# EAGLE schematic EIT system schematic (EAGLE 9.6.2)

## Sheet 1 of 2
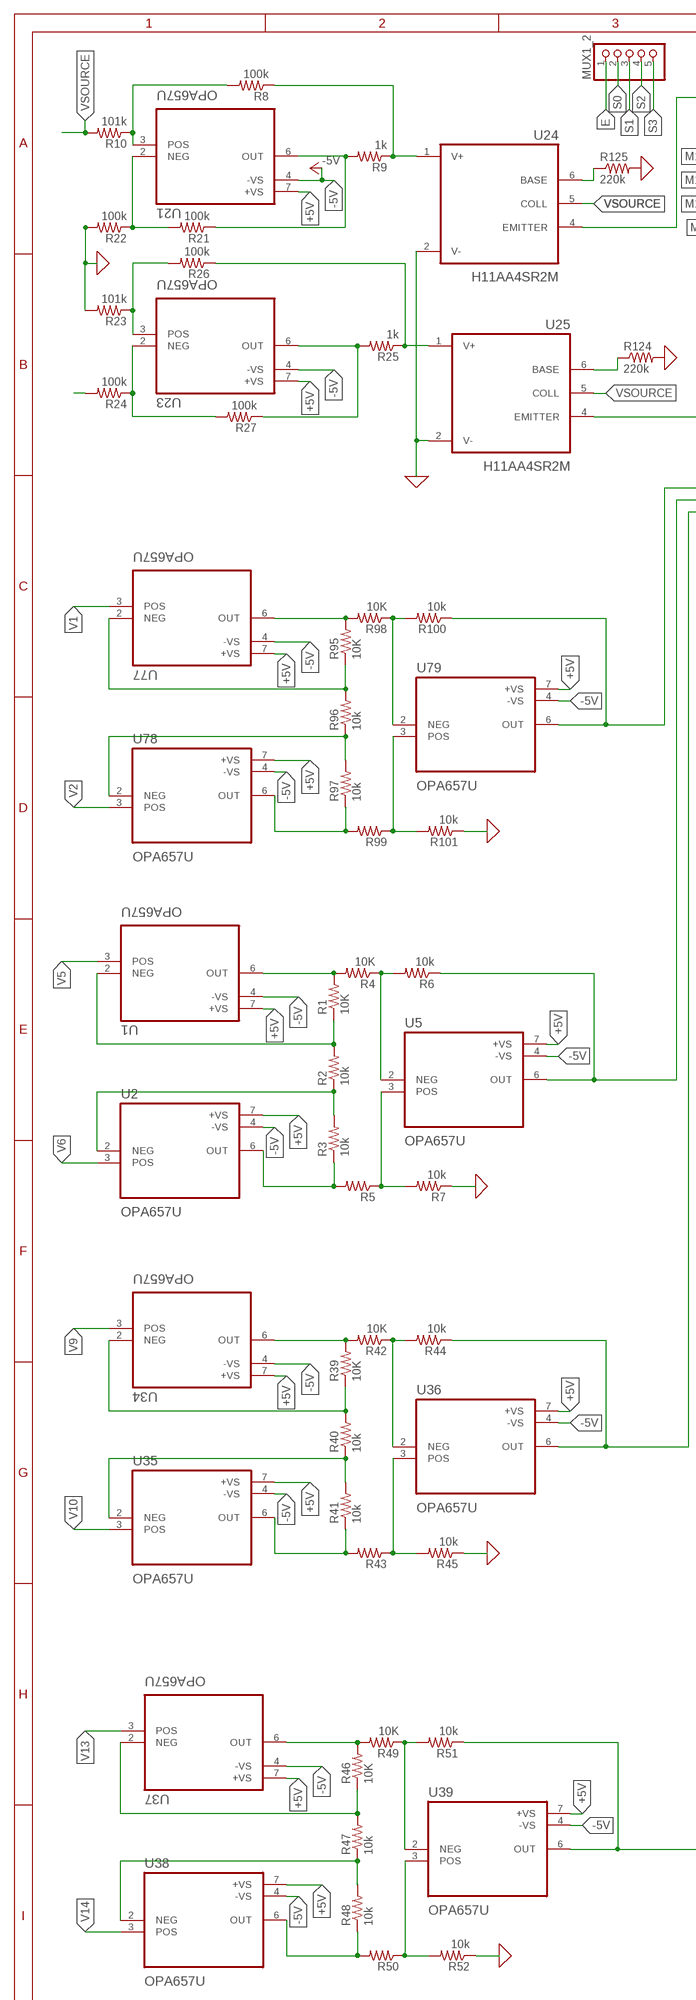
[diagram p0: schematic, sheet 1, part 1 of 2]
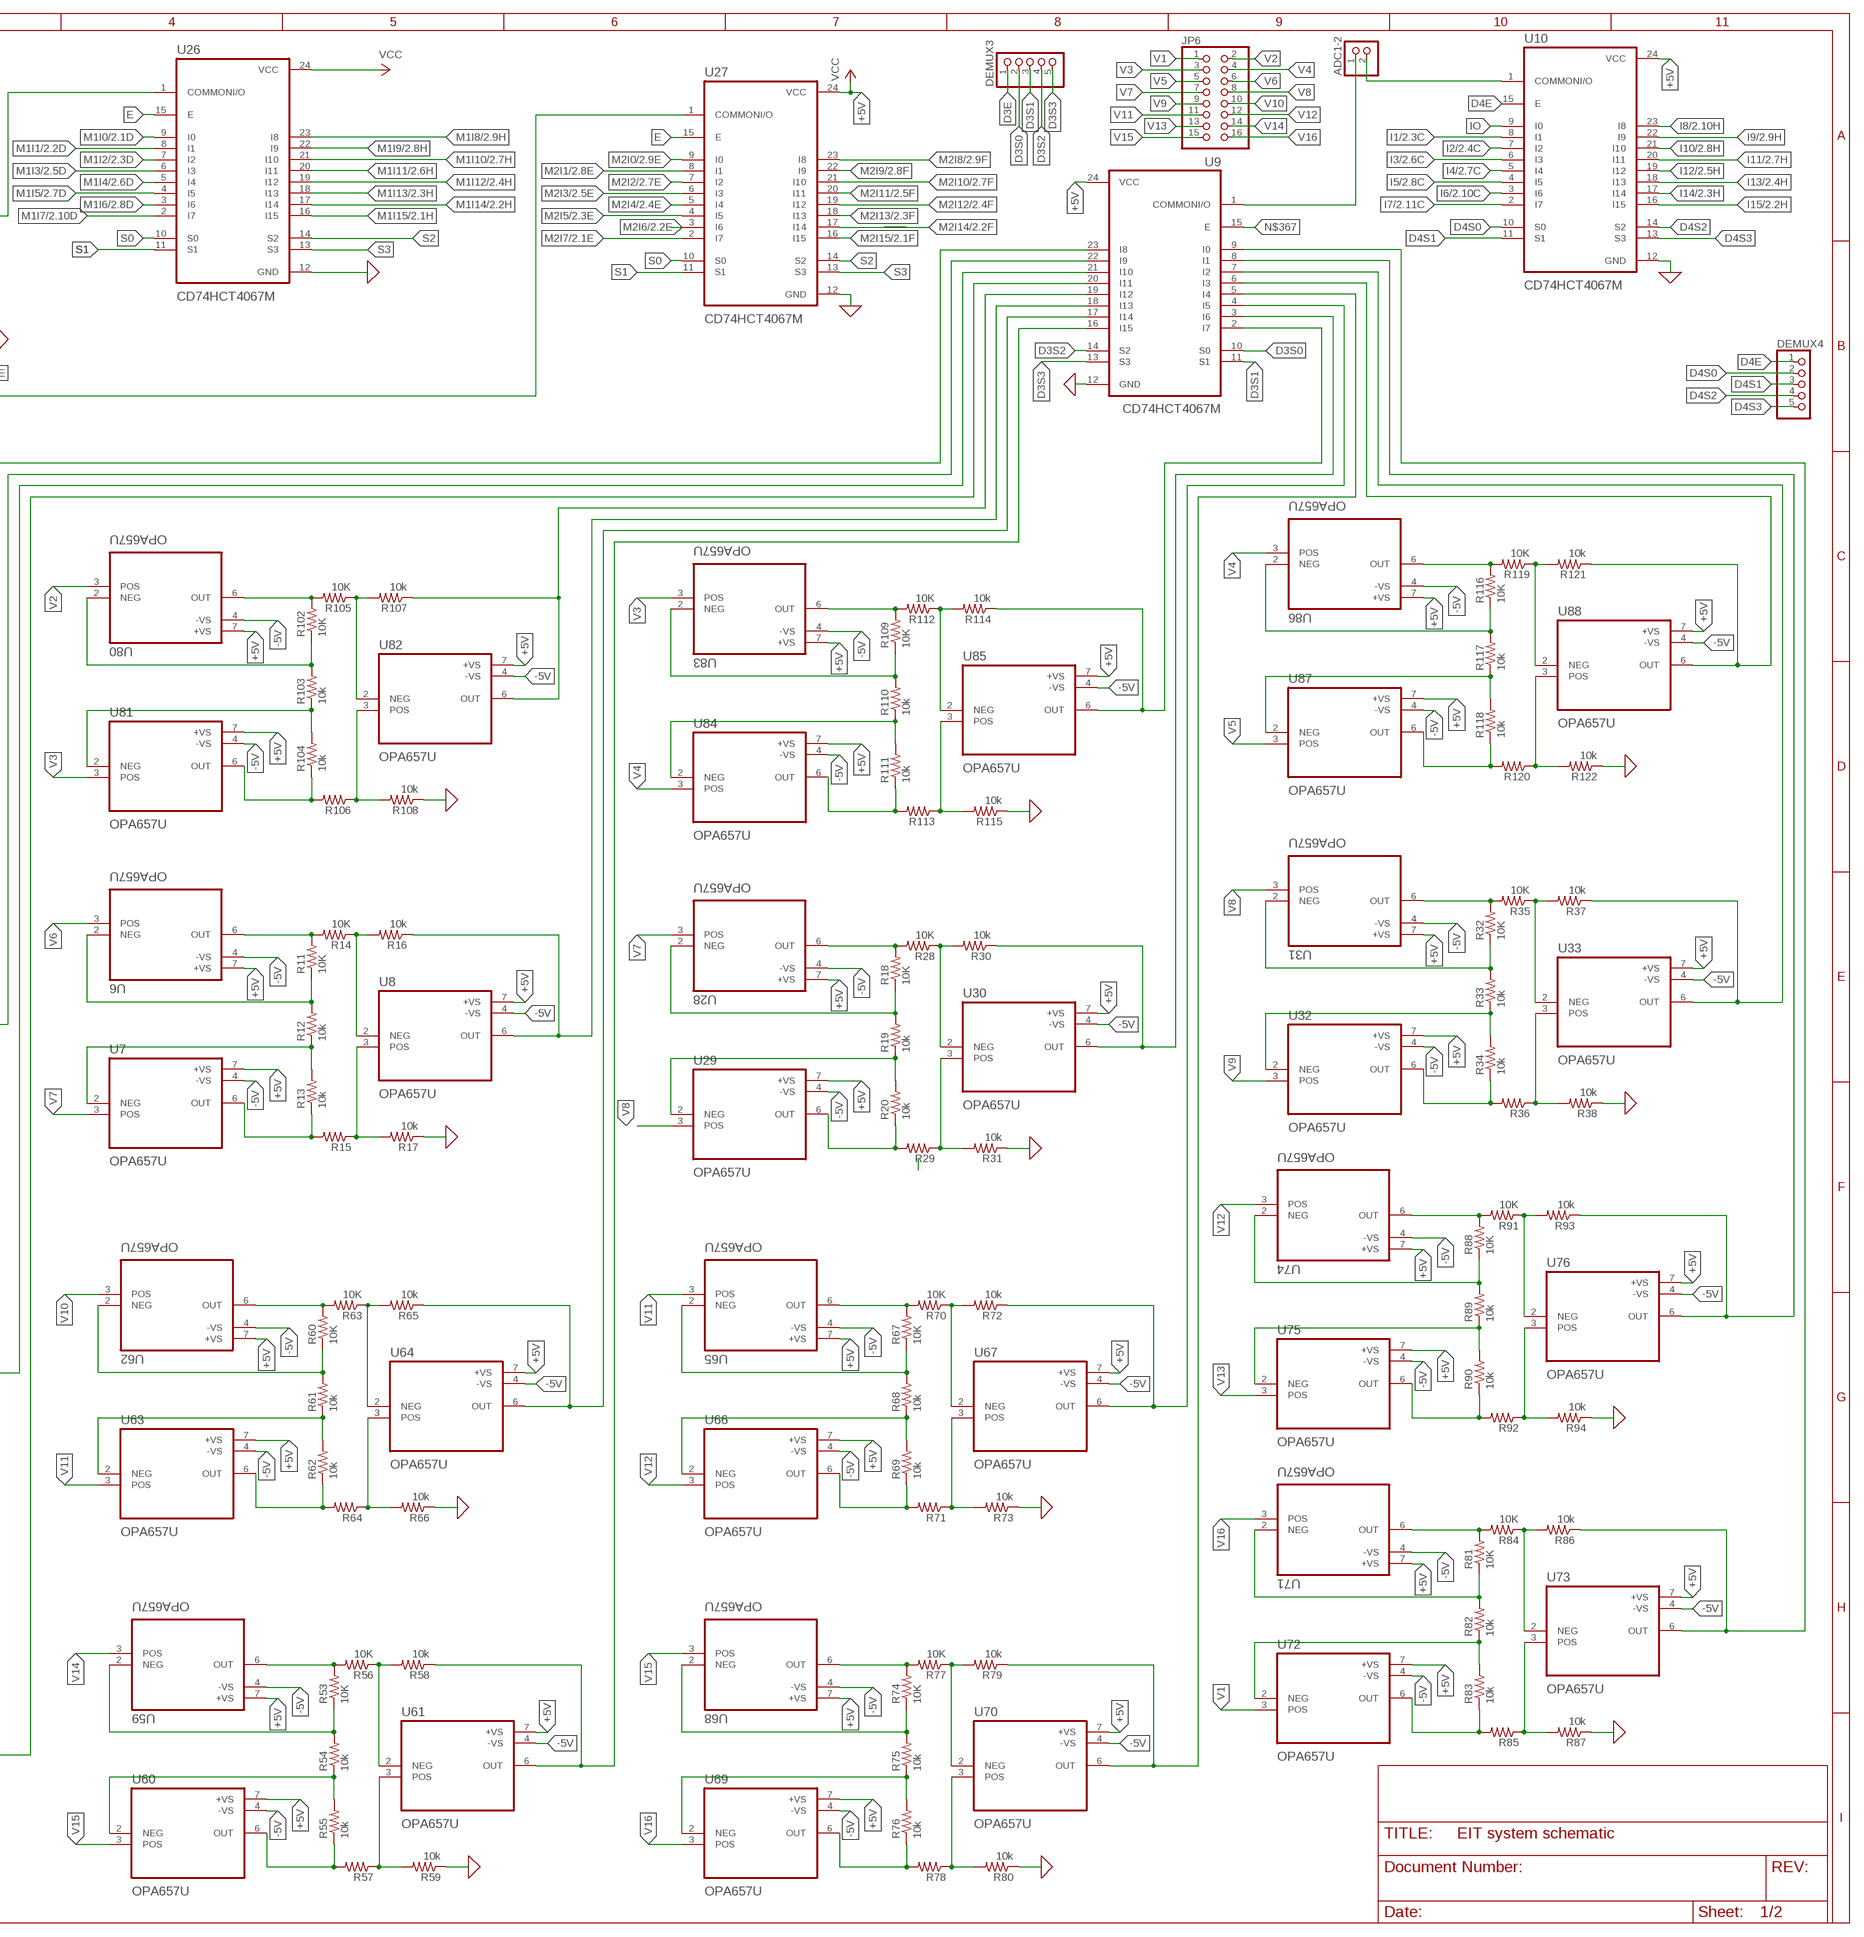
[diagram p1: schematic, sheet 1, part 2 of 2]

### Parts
ADC1-2  PINHD-1X2  [1X02]
DEMUX3  PINHD-1X5  [1X05]
DEMUX4  PINHD-1X5  [1X05]
JP6  PINHD-2X8  [2X08]
MUX1_2  PINHD-1X55X2MM  [1_05X2MM]
R1  10K  R-US_M0805  [M0805]
R2  10k  R-US_M0805  [M0805]
R3  10k  R-US_M0805  [M0805]
R4  10K  R-US_M0805  [M0805]
R5  R-US_M0805  [M0805]
R6  10k  R-US_M0805  [M0805]
R7  10k  R-US_M0805  [M0805]
R8  100k  R-US_M0805  [M0805]
R9  1k  R-US_M0805  [M0805]
R10  101k  R-US_M0805  [M0805]
R11  10K  R-US_M0805  [M0805]
R12  10k  R-US_M0805  [M0805]
R13  10k  R-US_M0805  [M0805]
R14  10K  R-US_M0805  [M0805]
R15  R-US_M0805  [M0805]
R16  10k  R-US_M0805  [M0805]
R17  10k  R-US_M0805  [M0805]
R18  10K  R-US_M0805  [M0805]
R19  10k  R-US_M0805  [M0805]
R20  10k  R-US_M0805  [M0805]
R21  100k  R-US_M0805  [M0805]
R22  100k  R-US_M0805  [M0805]
R23  101k  R-US_M0805  [M0805]
R24  100k  R-US_M0805  [M0805]
R25  1k  R-US_M0805  [M0805]
R26  100k  R-US_M0805  [M0805]
R27  100k  R-US_M0805  [M0805]
R28  10K  R-US_M0805  [M0805]
R29  R-US_M0805  [M0805]
R30  10k  R-US_M0805  [M0805]
R31  10k  R-US_M0805  [M0805]
R32  10K  R-US_M0805  [M0805]
R33  10k  R-US_M0805  [M0805]
R34  10k  R-US_M0805  [M0805]
R35  10K  R-US_M0805  [M0805]
R36  R-US_M0805  [M0805]
R37  10k  R-US_M0805  [M0805]
R38  10k  R-US_M0805  [M0805]
R39  10K  R-US_M0805  [M0805]
R40  10k  R-US_M0805  [M0805]
R41  10k  R-US_M0805  [M0805]
R42  10K  R-US_M0805  [M0805]
R43  R-US_M0805  [M0805]
R44  10k  R-US_M0805  [M0805]
R45  10k  R-US_M0805  [M0805]
R46  10K  R-US_M0805  [M0805]
R47  10k  R-US_M0805  [M0805]
R48  10k  R-US_M0805  [M0805]
R49  10K  R-US_M0805  [M0805]
R50  R-US_M0805  [M0805]
R51  10k  R-US_M0805  [M0805]
R52  10k  R-US_M0805  [M0805]
R53  10K  R-US_M0805  [M0805]
R54  10k  R-US_M0805  [M0805]
R55  10k  R-US_M0805  [M0805]
R56  10K  R-US_M0805  [M0805]
R57  R-US_M0805  [M0805]
R58  10k  R-US_M0805  [M0805]
R59  10k  R-US_M0805  [M0805]
R60  10K  R-US_M0805  [M0805]
R61  10k  R-US_M0805  [M0805]
R62  10k  R-US_M0805  [M0805]
R63  10K  R-US_M0805  [M0805]
R64  R-US_M0805  [M0805]
R65  10k  R-US_M0805  [M0805]
R66  10k  R-US_M0805  [M0805]
R67  10K  R-US_M0805  [M0805]
R68  10k  R-US_M0805  [M0805]
R69  10k  R-US_M0805  [M0805]
R70  10K  R-US_M0805  [M0805]
R71  R-US_M0805  [M0805]
R72  10k  R-US_M0805  [M0805]
R73  10k  R-US_M0805  [M0805]
R74  10K  R-US_M0805  [M0805]
R75  10k  R-US_M0805  [M0805]
R76  10k  R-US_M0805  [M0805]
R77  10K  R-US_M0805  [M0805]
R78  R-US_M0805  [M0805]
R79  10k  R-US_M0805  [M0805]
R80  10k  R-US_M0805  [M0805]
R81  10K  R-US_M0805  [M0805]
R82  10k  R-US_M0805  [M0805]
R83  10k  R-US_M0805  [M0805]
R84  10K  R-US_M0805  [M0805]
R85  R-US_M0805  [M0805]
R86  10k  R-US_M0805  [M0805]
R87  10k  R-US_M0805  [M0805]
R88  10K  R-US_M0805  [M0805]
R89  10k  R-US_M0805  [M0805]
R90  10k  R-US_M0805  [M0805]
R91  10K  R-US_M0805  [M0805]
R92  R-US_M0805  [M0805]
R93  10k  R-US_M0805  [M0805]
R94  10k  R-US_M0805  [M0805]
R95  10K  R-US_M0805  [M0805]
R96  10k  R-US_M0805  [M0805]
R97  10k  R-US_M0805  [M0805]
R98  10K  R-US_M0805  [M0805]
R99  R-US_M0805  [M0805]
R100  10k  R-US_M0805  [M0805]
R101  10k  R-US_M0805  [M0805]
R102  10K  R-US_M0805  [M0805]
R103  10k  R-US_M0805  [M0805]
R104  10k  R-US_M0805  [M0805]
R105  10K  R-US_M0805  [M0805]
R106  R-US_M0805  [M0805]
R107  10k  R-US_M0805  [M0805]
R108  10k  R-US_M0805  [M0805]
R109  10K  R-US_M0805  [M0805]
R110  10k  R-US_M0805  [M0805]
R111  10k  R-US_M0805  [M0805]
R112  10K  R-US_M0805  [M0805]
R113  R-US_M0805  [M0805]
R114  10k  R-US_M0805  [M0805]
R115  10k  R-US_M0805  [M0805]
R116  10K  R-US_M0805  [M0805]
R117  10k  R-US_M0805  [M0805]
R118  10k  R-US_M0805  [M0805]
R119  10K  R-US_M0805  [M0805]
R120  R-US_M0805  [M0805]
R121  10k  R-US_M0805  [M0805]
R122  10k  R-US_M0805  [M0805]
R124  220k  R-US_M0805  [M0805]
R125  220k  R-US_M0805  [M0805]
U1  OPA657U  [SOIC127P599X175-8N]
U2  OPA657U  [SOIC127P599X175-8N]
U5  OPA657U  [SOIC127P599X175-8N]
U6  OPA657U  [SOIC127P599X175-8N]
U7  OPA657U  [SOIC127P599X175-8N]
U8  OPA657U  [SOIC127P599X175-8N]
U9  CD74HCT4067M  [SOIC127P1030X265-24N]
U10  CD74HCT4067M  [SOIC127P1030X265-24N]
U21  OPA657U  [SOIC127P599X175-8N]
U23  OPA657U  [SOIC127P599X175-8N]
U24  H11AA4SR2M  [OPTOCOUPLER_H11F3SR2M]
U25  H11AA4SR2M  [OPTOCOUPLER_H11F3SR2M]
U26  CD74HCT4067M  [SOIC127P1030X265-24N]
U27  CD74HCT4067M  [SOIC127P1030X265-24N]
U28  OPA657U  [SOIC127P599X175-8N]
U29  OPA657U  [SOIC127P599X175-8N]
U30  OPA657U  [SOIC127P599X175-8N]
U31  OPA657U  [SOIC127P599X175-8N]
U32  OPA657U  [SOIC127P599X175-8N]
U33  OPA657U  [SOIC127P599X175-8N]
U34  OPA657U  [SOIC127P599X175-8N]
U35  OPA657U  [SOIC127P599X175-8N]
U36  OPA657U  [SOIC127P599X175-8N]
U37  OPA657U  [SOIC127P599X175-8N]
U38  OPA657U  [SOIC127P599X175-8N]
U39  OPA657U  [SOIC127P599X175-8N]
U59  OPA657U  [SOIC127P599X175-8N]
U60  OPA657U  [SOIC127P599X175-8N]
U61  OPA657U  [SOIC127P599X175-8N]
U62  OPA657U  [SOIC127P599X175-8N]
U63  OPA657U  [SOIC127P599X175-8N]
U64  OPA657U  [SOIC127P599X175-8N]
U65  OPA657U  [SOIC127P599X175-8N]
U66  OPA657U  [SOIC127P599X175-8N]
U67  OPA657U  [SOIC127P599X175-8N]
U68  OPA657U  [SOIC127P599X175-8N]
U69  OPA657U  [SOIC127P599X175-8N]
U70  OPA657U  [SOIC127P599X175-8N]
U71  OPA657U  [SOIC127P599X175-8N]
U72  OPA657U  [SOIC127P599X175-8N]
U73  OPA657U  [SOIC127P599X175-8N]
U74  OPA657U  [SOIC127P599X175-8N]
U75  OPA657U  [SOIC127P599X175-8N]
U76  OPA657U  [SOIC127P599X175-8N]
U77  OPA657U  [SOIC127P599X175-8N]
U78  OPA657U  [SOIC127P599X175-8N]
U79  OPA657U  [SOIC127P599X175-8N]
U80  OPA657U  [SOIC127P599X175-8N]
U81  OPA657U  [SOIC127P599X175-8N]
U82  OPA657U  [SOIC127P599X175-8N]
U83  OPA657U  [SOIC127P599X175-8N]
U84  OPA657U  [SOIC127P599X175-8N]
U85  OPA657U  [SOIC127P599X175-8N]
U86  OPA657U  [SOIC127P599X175-8N]
U87  OPA657U  [SOIC127P599X175-8N]
U88  OPA657U  [SOIC127P599X175-8N]

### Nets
0: R7.1 R17.1 R22.2 R23.2 R31.1 R38.1 R45.1 R52.1 R59.1 R66.1 R73.1 R80.1 R87.1 R94.1 R101.1 R108.1 R115.1 R122.1 R124.2 R125.2 U9.12(GND) U10.12(GND) U24.2(V-) U25.2(V-) U26.12(GND) U27.12(GND) ; supply symbol labelled GND ; also sheet 2
+5V: U27.24(VCC) ; supply symbol labelled VCC
-5V: U21.4(-VS)
D3E: DEMUX3.1
D3S0: DEMUX3.2 U9.10(S0)
D3S1: DEMUX3.3 U9.11(S1)
D3S2: DEMUX3.4 U9.14(S2)
D3S3: DEMUX3.5 U9.13(S3)
D4E: DEMUX4.1
D4S0: DEMUX4.2
D4S1: DEMUX4.3
D4S2: DEMUX4.4
D4S3: DEMUX4.5
E: MUX1_2.1 U26.15(E)
I1: U10.8(I1) ; also sheet 2
I2: U10.7(I2) ; also sheet 2
I3: U10.6(I3) ; also sheet 2
I4: U10.5(I4) ; also sheet 2
I5: U10.4(I5) ; also sheet 2
I6: U10.3(I6) ; also sheet 2
I7: U10.2(I7) ; also sheet 2
I8: U10.23(I8) ; also sheet 2
I9: U10.22(I9) ; also sheet 2
I10: U10.21(I10) ; also sheet 2
I11: U10.20(I11) ; also sheet 2
I12: U10.19(I12) ; also sheet 2
I13: U10.18(I13) ; also sheet 2
I14: U10.17(I14) ; also sheet 2
I15: U10.16(I15) ; also sheet 2
IO: U10.9(I0)
M1I0: U26.9(I0) ; also sheet 2
M1I1: U26.8(I1) ; also sheet 2
M1I2: U26.7(I2) ; also sheet 2
M1I3: U26.6(I3) ; also sheet 2
M1I4: U26.5(I4) ; also sheet 2
M1I5: U26.4(I5) ; also sheet 2
M1I6: U26.3(I6) ; also sheet 2
M1I7: U26.2(I7) ; also sheet 2
M1I8: U26.23(I8) ; also sheet 2
M1I9: U26.22(I9) ; also sheet 2
M1I10: U26.21(I10) ; also sheet 2
M1I11: U26.20(I11) ; also sheet 2
M1I12: U26.19(I12) ; also sheet 2
M1I13: U26.18(I13) ; also sheet 2
M1I14: U26.17(I14) ; also sheet 2
M1I15: U26.16(I15) ; also sheet 2
M2I0: U27.9(I0) ; also sheet 2
M2I1: U27.8(I1) ; also sheet 2
M2I2: U27.7(I2) ; also sheet 2
M2I3: U27.6(I3) ; also sheet 2
M2I4: U27.5(I4) ; also sheet 2
M2I5: U27.4(I5) ; also sheet 2
M2I6: U27.3(I6) ; also sheet 2
M2I7: U27.2(I7) ; also sheet 2
M2I8: U27.23(I8) ; also sheet 2
M2I9: U27.22(I9) ; also sheet 2
M2I10: U27.21(I10) ; also sheet 2
M2I11: U27.20(I11) ; also sheet 2
M2I12: U27.19(I12) ; also sheet 2
M2I13: U27.18(I13) ; also sheet 2
M2I14: U27.17(I14) ; also sheet 2
M2I15: U27.16(I15) ; also sheet 2
N$1: U9.24(VCC)
N$3: U1.4(-VS)
N$4: U1.7(+VS)
N$5: U2.4(-VS)
N$6: U2.7(+VS)
N$7: U5.4(-VS)
N$8: U5.7(+VS)
N$9: U23.4(-VS)
N$10: U23.7(+VS)
N$11: U25.4(EMITTER) U27.1(COMMONI/O)
N$12: ADC1-2.2 U10.1(COMMONI/O)
N$13: R124.1 U25.6(BASE)
N$18: R2.1 R3.2 U2.2(NEG)
N$20: R1.1 R2.2 U1.2(NEG)
N$22: R3.1 R5.2 U2.6(OUT)
N$24: R5.1 R7.2 U5.3(POS)
N$28: R1.2 R4.2 U1.6(OUT)
N$29: R4.1 R6.2 U5.2(NEG)
N$34: R6.1 U5.6(OUT) U9.22(I9)
N$38: R125.1 U24.6(BASE)
N$79: U6.4(-VS)
N$91: U6.7(+VS)
N$95: U7.4(-VS)
N$99: U7.7(+VS)
N$103: U8.4(-VS)
N$107: U8.7(+VS)
N$111: R37.1 U9.7(I2) U33.6(OUT)
N$121: R8.2 R10.1 U21.3(POS)
N$122: R21.2 R22.1 U21.2(NEG)
N$123: R9.2 R21.1 U21.6(OUT)
N$124: R8.1 R9.1 U24.1(V+)
N$125: R23.1 R26.2 U23.3(POS)
N$126: R24.1 R27.2 U23.2(NEG)
N$127: R25.2 R27.1 U23.6(OUT)
N$128: R25.1 R26.1 U25.1(V+)
N$129: R24.2
N$130: U25.5(COLL)
N$131: U24.4(EMITTER) U26.1(COMMONI/O)
N$132: U80.4(-VS)
N$133: U27.10(S0)
N$134: U27.11(S1)
N$135: U27.15(E)
N$136: U27.14(S2)
N$137: U27.13(S3)
N$138: R93.1 U9.8(I1) U76.6(OUT)
N$139: R12.1 R13.2 U7.2(NEG)
N$140: R11.1 R12.2 U6.2(NEG)
N$141: R13.1 R15.2 U7.6(OUT)
N$142: R15.1 R17.2 U8.3(POS)
N$143: R11.2 R14.2 U6.6(OUT)
N$144: R14.1 R16.2 U8.2(NEG)
N$145: R16.1 U8.6(OUT) U9.18(I13)
N$146: U28.4(-VS)
N$147: U28.7(+VS)
N$148: U29.4(-VS)
N$149: U29.7(+VS)
N$150: U30.4(-VS)
N$151: U30.7(+VS)
N$152: R86.1 U9.9(I0) U73.6(OUT)
N$153: U10.24(VCC)
N$154: R19.1 R20.2 U29.2(NEG)
N$155: R18.1 R19.2 U28.2(NEG)
N$156: R20.1 R29.2 U29.6(OUT)
N$157: R29.1 R31.2 U30.3(POS)
N$158: R18.2 R28.2 U28.6(OUT)
N$159: R28.1 R30.2 U30.2(NEG)
N$160: R30.1 U9.3(I6) U30.6(OUT)
N$161: U31.4(-VS)
N$162: U31.7(+VS)
N$163: U32.4(-VS)
N$164: U32.7(+VS)
N$165: U33.4(-VS)
N$166: U33.7(+VS)
N$167: U10.10(S0)
N$168: U10.11(S1)
N$169: R33.1 R34.2 U32.2(NEG)
N$170: R32.1 R33.2 U31.2(NEG)
N$171: R34.1 R36.2 U32.6(OUT)
N$172: R36.1 R38.2 U33.3(POS)
N$173: R32.2 R35.2 U31.6(OUT)
N$174: R35.1 R37.2 U33.2(NEG)
N$175: U10.13(S3)
N$176: U34.4(-VS)
N$177: U34.7(+VS)
N$178: U35.4(-VS)
N$179: U35.7(+VS)
N$180: U36.4(-VS)
N$181: U36.7(+VS)
N$182: U10.14(S2)
N$184: R40.1 R41.2 U35.2(NEG)
N$185: R39.1 R40.2 U34.2(NEG)
N$186: R41.1 R43.2 U35.6(OUT)
N$187: R43.1 R45.2 U36.3(POS)
N$188: R39.2 R42.2 U34.6(OUT)
N$189: R42.1 R44.2 U36.2(NEG)
N$190: R44.1 U9.21(I10) U36.6(OUT)
N$191: U37.4(-VS)
N$192: U37.7(+VS)
N$193: U38.4(-VS)
N$194: U38.7(+VS)
N$195: U39.4(-VS)
N$196: U39.7(+VS)
N$199: R47.1 R48.2 U38.2(NEG)
N$200: R46.1 R47.2 U37.2(NEG)
N$201: R48.1 R50.2 U38.6(OUT)
N$202: R50.1 R52.2 U39.3(POS)
N$203: R46.2 R49.2 U37.6(OUT)
N$204: R49.1 R51.2 U39.2(NEG)
N$205: R51.1 U9.20(I11) U39.6(OUT)
N$206: U59.4(-VS)
N$207: U59.7(+VS)
N$208: U60.4(-VS)
N$209: U60.7(+VS)
N$210: U61.4(-VS)
N$211: U61.7(+VS)
N$214: R54.1 R55.2 U60.2(NEG)
N$215: R53.1 R54.2 U59.2(NEG)
N$216: R55.1 R57.2 U60.6(OUT)
N$217: R57.1 R59.2 U61.3(POS)
N$218: R53.2 R56.2 U59.6(OUT)
N$219: R56.1 R58.2 U61.2(NEG)
N$220: R58.1 U9.16(I15) U61.6(OUT)
N$221: U62.4(-VS)
N$222: U62.7(+VS)
N$223: U63.4(-VS)
N$224: U63.7(+VS)
N$225: U64.4(-VS)
N$226: U64.7(+VS)
N$229: R61.1 R62.2 U63.2(NEG)
N$230: R60.1 R61.2 U62.2(NEG)
N$231: R62.1 R64.2 U63.6(OUT)
N$232: R64.1 R66.2 U64.3(POS)
N$233: R60.2 R63.2 U62.6(OUT)
N$234: R63.1 R65.2 U64.2(NEG)
N$235: R65.1 U9.17(I14) U64.6(OUT)
N$236: U65.4(-VS)
N$237: U65.7(+VS)
N$238: U66.4(-VS)
N$239: U66.7(+VS)
N$240: U67.4(-VS)
N$241: U67.7(+VS)
N$244: R68.1 R69.2 U66.2(NEG)
N$245: R67.1 R68.2 U65.2(NEG)
N$246: R69.1 R71.2 U66.6(OUT)
N$247: R71.1 R73.2 U67.3(POS)
N$248: R67.2 R70.2 U65.6(OUT)
N$249: R70.1 R72.2 U67.2(NEG)
N$250: R72.1 U9.4(I5) U67.6(OUT)
N$251: U68.4(-VS)
N$252: U68.7(+VS)
N$253: U69.4(-VS)
N$254: U69.7(+VS)
N$255: U70.4(-VS)
N$256: U70.7(+VS)
N$259: R75.1 R76.2 U69.2(NEG)
N$260: R74.1 R75.2 U68.2(NEG)
N$261: R76.1 R78.2 U69.6(OUT)
N$262: R78.1 R80.2 U70.3(POS)
N$263: R74.2 R77.2 U68.6(OUT)
N$264: R77.1 R79.2 U70.2(NEG)
N$265: R79.1 U9.5(I4) U70.6(OUT)
N$266: U71.4(-VS)
N$267: U71.7(+VS)
N$268: U72.4(-VS)
N$269: U72.7(+VS)
N$270: U73.4(-VS)
N$271: U73.7(+VS)
N$274: R82.1 R83.2 U72.2(NEG)
N$275: R81.1 R82.2 U71.2(NEG)
N$276: R83.1 R85.2 U72.6(OUT)
N$277: R85.1 R87.2 U73.3(POS)
N$278: R81.2 R84.2 U71.6(OUT)
N$279: R84.1 R86.2 U73.2(NEG)
N$281: U74.4(-VS)
N$282: U74.7(+VS)
N$283: U75.4(-VS)
N$284: U75.7(+VS)
N$285: U76.4(-VS)
N$286: U76.7(+VS)
N$289: R89.1 R90.2 U75.2(NEG)
N$290: R88.1 R89.2 U74.2(NEG)
N$291: R90.1 R92.2 U75.6(OUT)
N$292: R92.1 R94.2 U76.3(POS)
N$293: R88.2 R91.2 U74.6(OUT)
N$294: R91.1 R93.2 U76.2(NEG)
N$296: U77.4(-VS)
N$297: U77.7(+VS)
N$298: U21.7(+VS)
N$299: U78.4(-VS)
N$300: U78.7(+VS)
N$301: U79.4(-VS)
N$302: U79.7(+VS)
N$305: R96.1 R97.2 U78.2(NEG)
N$306: R95.1 R96.2 U77.2(NEG)
N$307: R97.1 R99.2 U78.6(OUT)
N$308: R99.1 R101.2 U79.3(POS)
N$309: R95.2 R98.2 U77.6(OUT)
N$310: R98.1 R100.2 U79.2(NEG)
N$311: R100.1 U9.23(I8) U79.6(OUT)
N$312: U80.7(+VS)
N$313: U81.4(-VS)
N$314: U81.7(+VS)
N$315: U82.4(-VS)
N$316: U82.7(+VS)
N$319: R103.1 R104.2 U81.2(NEG)
N$320: R102.1 R103.2 U80.2(NEG)
N$321: R104.1 R106.2 U81.6(OUT)
N$322: R106.1 R108.2 U82.3(POS)
N$323: R102.2 R105.2 U80.6(OUT)
N$324: R105.1 R107.2 U82.2(NEG)
N$325: R107.1 U9.19(I12) U82.6(OUT)
N$326: U83.4(-VS)
N$327: U83.7(+VS)
N$328: U84.4(-VS)
N$329: U84.7(+VS)
N$330: U85.4(-VS)
N$331: U85.7(+VS)
N$334: R110.1 R111.2 U84.2(NEG)
N$335: R109.1 R110.2 U83.2(NEG)
N$336: R111.1 R113.2 U84.6(OUT)
N$337: R113.1 R115.2 U85.3(POS)
N$338: R109.2 R112.2 U83.6(OUT)
N$339: R112.1 R114.2 U85.2(NEG)
N$340: R114.1 U9.2(I7) U85.6(OUT)
N$341: U86.4(-VS)
N$342: U86.7(+VS)
N$343: U87.4(-VS)
N$344: U87.7(+VS)
N$345: U88.4(-VS)
N$346: U88.7(+VS)
N$349: R117.1 R118.2 U87.2(NEG)
N$350: R116.1 R117.2 U86.2(NEG)
N$351: R118.1 R120.2 U87.6(OUT)
N$352: R120.1 R122.2 U88.3(POS)
N$353: R116.2 R119.2 U86.6(OUT)
N$354: R119.1 R121.2 U88.2(NEG)
N$355: R121.1 U9.6(I3) U88.6(OUT)
N$361: ADC1-2.1 U9.1(COMMONI/O)
N$367: U9.15(E)
S0: MUX1_2.2 U26.10(S0)
S1: MUX1_2.3 U26.11(S1)
S2: MUX1_2.4 U26.14(S2)
S3: MUX1_2.5 U26.13(S3)
V1: JP6.1 U72.3(POS) U77.3(POS)
V2: JP6.2 U78.3(POS) U80.3(POS)
V3: JP6.3 U81.3(POS) U83.3(POS)
V4: JP6.4 U84.3(POS) U86.3(POS)
V5: JP6.5 U1.3(POS) U87.3(POS)
V6: JP6.6 U2.3(POS) U6.3(POS)
V7: JP6.7 U7.3(POS) U28.3(POS)
V8: JP6.8 U29.3(POS) U31.3(POS)
V9: JP6.9 U32.3(POS) U34.3(POS)
V10: JP6.10 U35.3(POS) U62.3(POS)
V11: JP6.11 U63.3(POS) U65.3(POS)
V12: JP6.12 U66.3(POS) U74.3(POS)
V13: JP6.13 U37.3(POS) U75.3(POS)
V14: JP6.14 U38.3(POS) U59.3(POS)
V15: JP6.15 U60.3(POS) U68.3(POS)
V16: JP6.16 U69.3(POS) U71.3(POS)
VCC: U26.24(VCC)
VSOURCE: R10.2 U24.5(COLL)
Unconnected: U10.15(E)

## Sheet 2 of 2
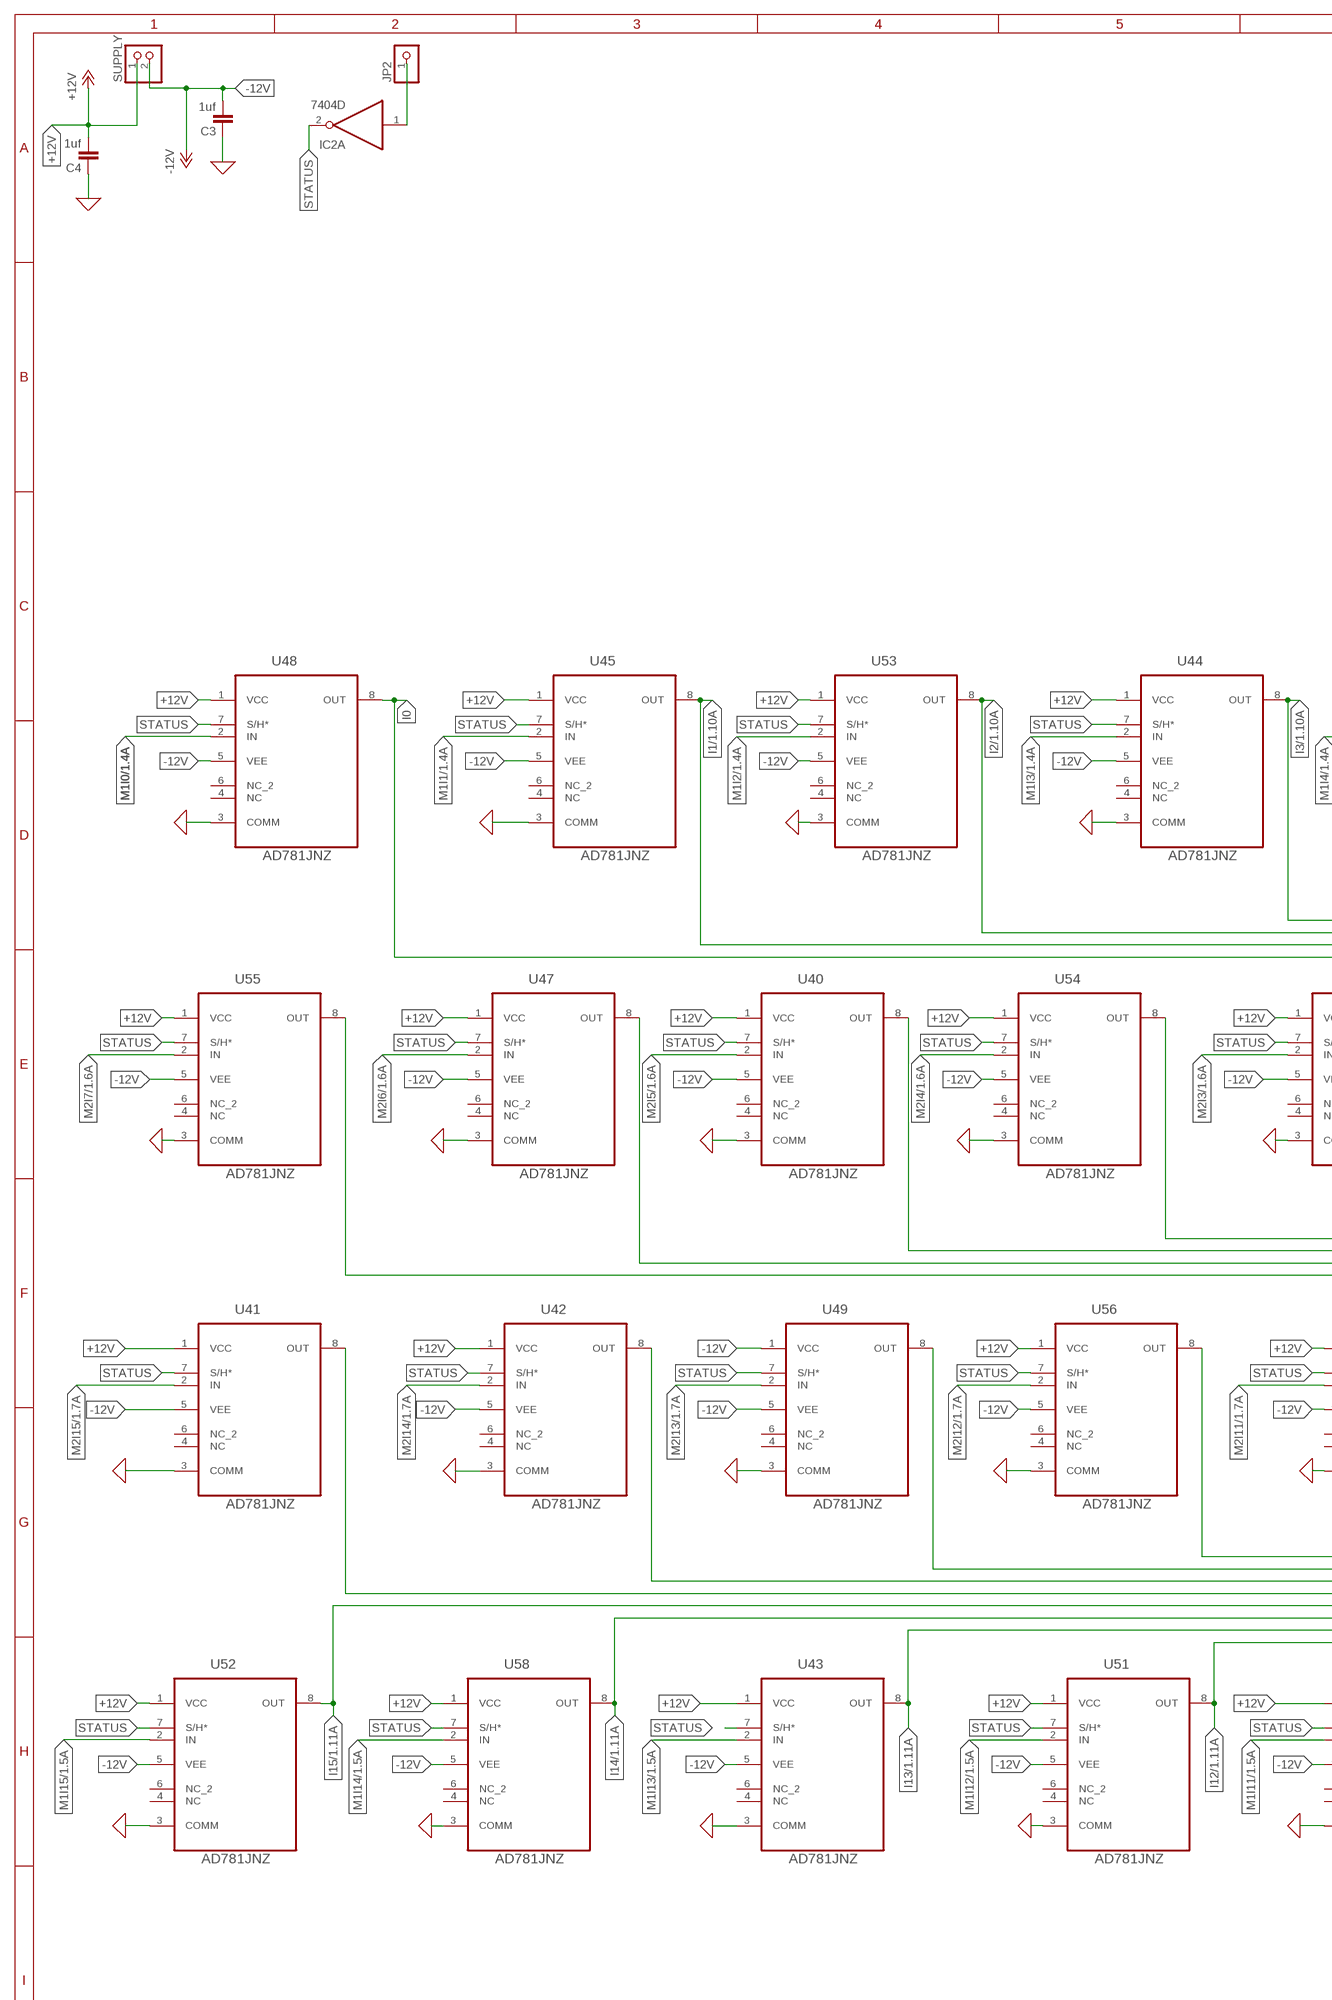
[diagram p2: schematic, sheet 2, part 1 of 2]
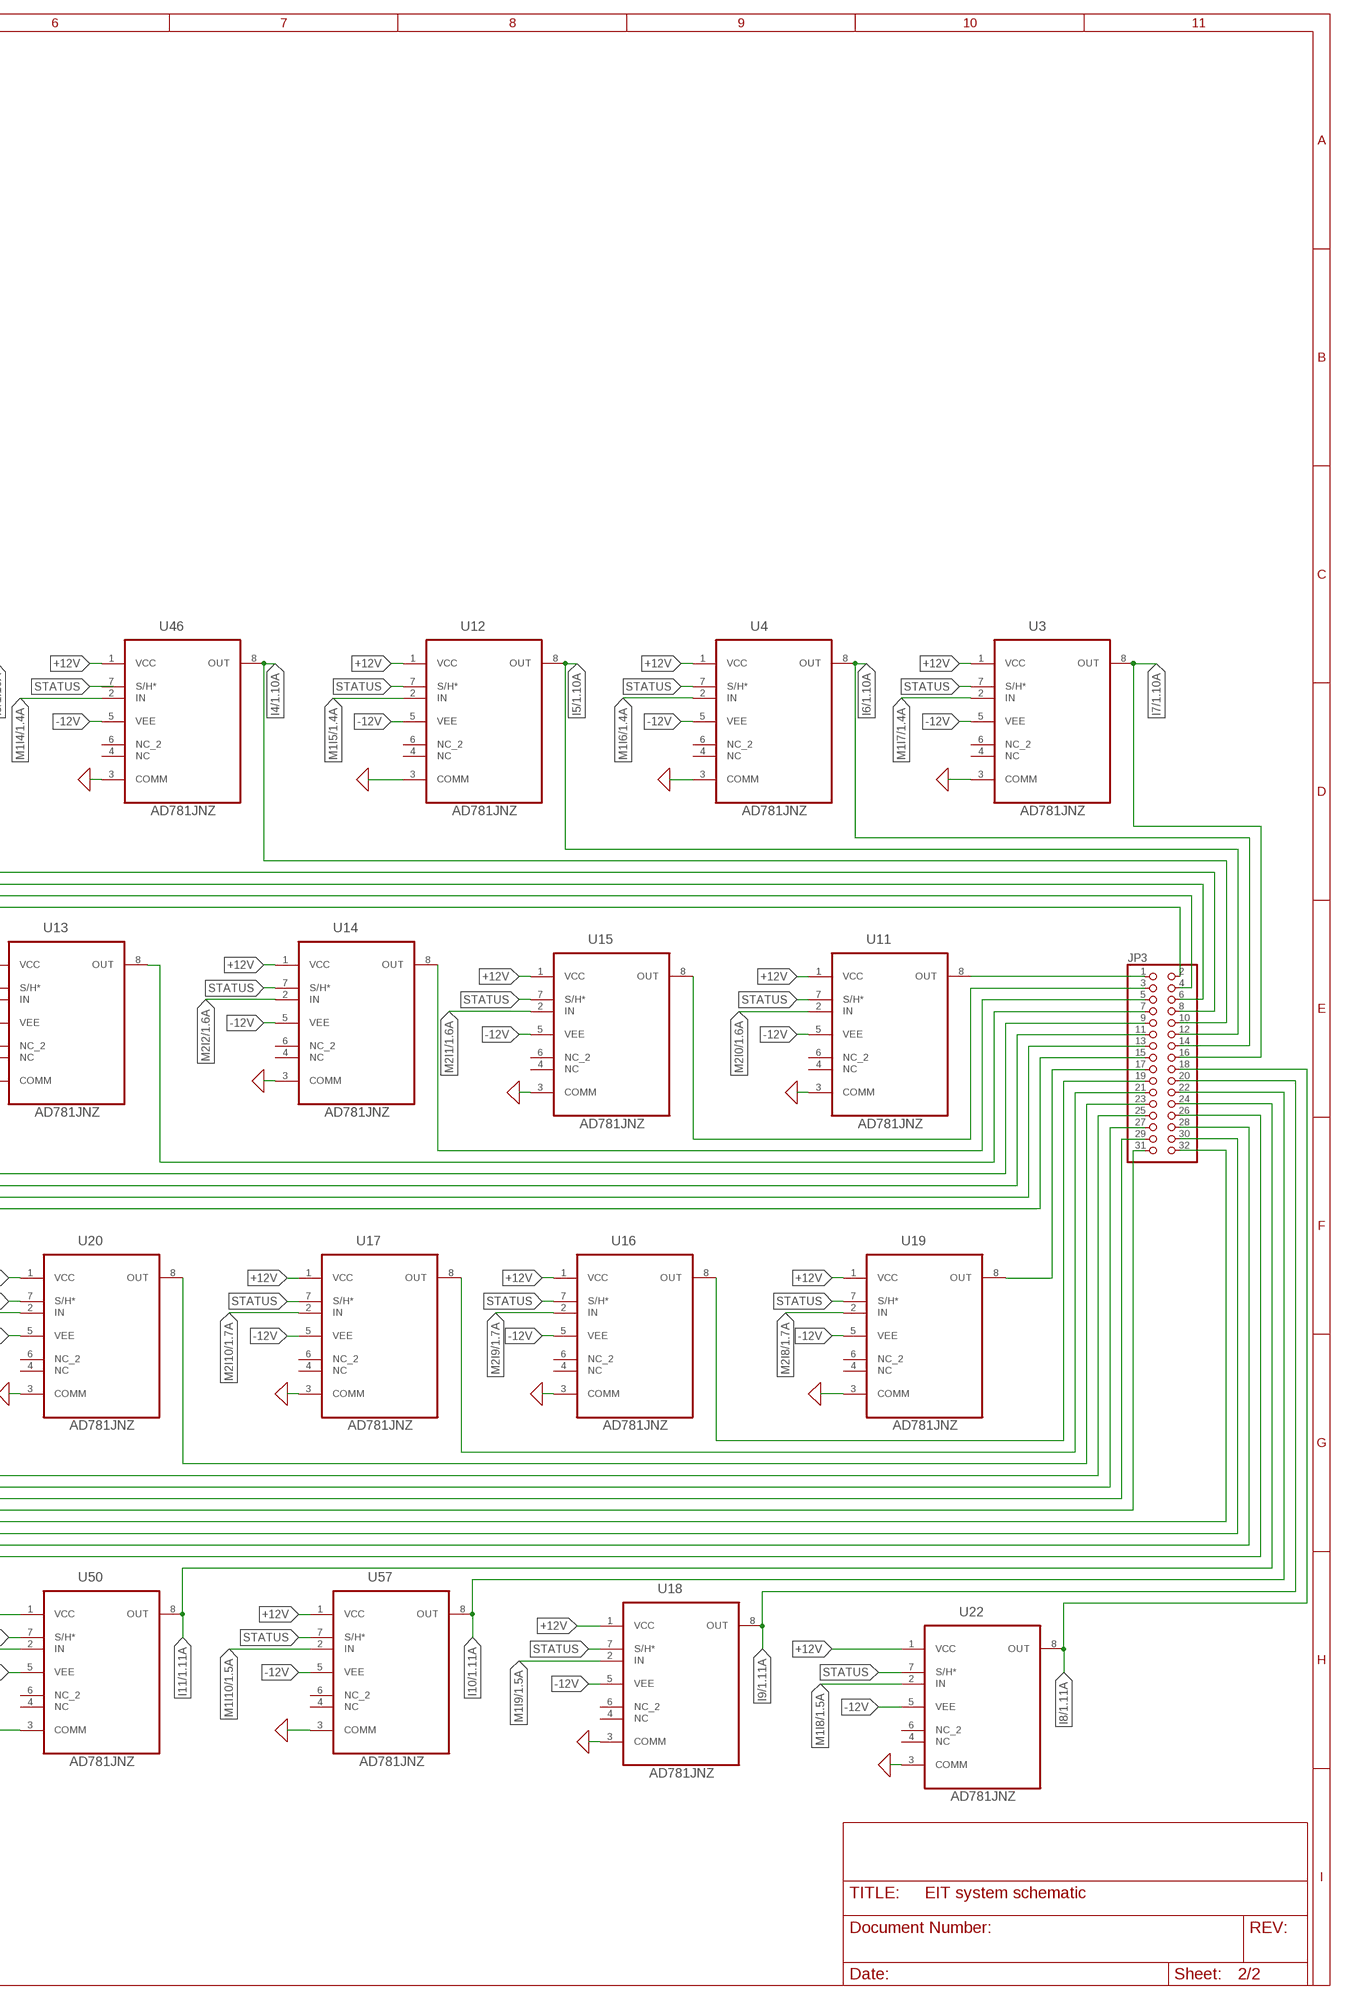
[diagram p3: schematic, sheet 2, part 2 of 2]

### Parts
C3  1uf  C-EUC0805  [C0805]
C4  1uf  C-EUC0805  [C0805]
IC2  7404D  [SO14]
JP2  PINHD-1X1  [1X01]
JP3  PINHD-2X16  [2X16]
SUPPLY  PINHD-1X2  [1X02]
U3  AD781JNZ  [DIP254P762X533-8]
U4  AD781JNZ  [DIP254P762X533-8]
U11  AD781JNZ  [DIP254P762X533-8]
U12  AD781JNZ  [DIP254P762X533-8]
U13  AD781JNZ  [DIP254P762X533-8]
U14  AD781JNZ  [DIP254P762X533-8]
U15  AD781JNZ  [DIP254P762X533-8]
U16  AD781JNZ  [DIP254P762X533-8]
U17  AD781JNZ  [DIP254P762X533-8]
U18  AD781JNZ  [DIP254P762X533-8]
U19  AD781JNZ  [DIP254P762X533-8]
U20  AD781JNZ  [DIP254P762X533-8]
U22  AD781JNZ  [DIP254P762X533-8]
U40  AD781JNZ  [DIP254P762X533-8]
U41  AD781JNZ  [DIP254P762X533-8]
U42  AD781JNZ  [DIP254P762X533-8]
U43  AD781JNZ  [DIP254P762X533-8]
U44  AD781JNZ  [DIP254P762X533-8]
U45  AD781JNZ  [DIP254P762X533-8]
U46  AD781JNZ  [DIP254P762X533-8]
U47  AD781JNZ  [DIP254P762X533-8]
U48  AD781JNZ  [DIP254P762X533-8]
U49  AD781JNZ  [DIP254P762X533-8]
U50  AD781JNZ  [DIP254P762X533-8]
U51  AD781JNZ  [DIP254P762X533-8]
U52  AD781JNZ  [DIP254P762X533-8]
U53  AD781JNZ  [DIP254P762X533-8]
U54  AD781JNZ  [DIP254P762X533-8]
U55  AD781JNZ  [DIP254P762X533-8]
U56  AD781JNZ  [DIP254P762X533-8]
U57  AD781JNZ  [DIP254P762X533-8]
U58  AD781JNZ  [DIP254P762X533-8]

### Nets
0: C3.1 C4.1 U3.3(COMM) U4.3(COMM) U11.3(COMM) U12.3(COMM) U13.3(COMM) U14.3(COMM) U15.3(COMM) U16.3(COMM) U17.3(COMM) U18.3(COMM) U19.3(COMM) U20.3(COMM) U22.3(COMM) U40.3(COMM) U41.3(COMM) U42.3(COMM) U43.3(COMM) U44.3(COMM) U45.3(COMM) U46.3(COMM) U47.3(COMM) U48.3(COMM) U49.3(COMM) U50.3(COMM) U51.3(COMM) U52.3(COMM) U53.3(COMM) U54.3(COMM) U55.3(COMM) U56.3(COMM) U57.3(COMM) U58.3(COMM) ; supply symbol labelled GND ; also sheet 1
+12V: C4.2 SUPPLY.1 U13.1(VCC) U14.1(VCC) U17.1(VCC) U20.1(VCC) U40.1(VCC) U41.1(VCC) U42.1(VCC) U44.1(VCC) U45.1(VCC) U46.1(VCC) U47.1(VCC) U48.1(VCC) U53.1(VCC) U54.1(VCC) U55.1(VCC) U56.1(VCC)
-12V: C3.2 SUPPLY.2 U13.5(VEE) U14.5(VEE) U17.5(VEE) U20.5(VEE) U40.5(VEE) U41.5(VEE) U42.5(VEE) U44.5(VEE) U45.5(VEE) U46.5(VEE) U47.5(VEE) U48.5(VEE) U49.1(VCC) U53.5(VEE) U54.5(VEE) U55.5(VEE) U56.5(VEE)
I0: JP3.2 U48.8(OUT)
I1: JP3.4 U45.8(OUT) ; also sheet 1
I2: JP3.6 U53.8(OUT) ; also sheet 1
I3: JP3.8 U44.8(OUT) ; also sheet 1
I4: JP3.10 U46.8(OUT) ; also sheet 1
I5: JP3.12 U12.8(OUT) ; also sheet 1
I6: JP3.14 U4.8(OUT) ; also sheet 1
I7: JP3.16 U3.8(OUT) ; also sheet 1
I8: JP3.18 U22.8(OUT) ; also sheet 1
I9: JP3.20 U18.8(OUT) ; also sheet 1
I10: JP3.22 U57.8(OUT) ; also sheet 1
I11: JP3.24 U50.8(OUT) ; also sheet 1
I12: JP3.26 U51.8(OUT) ; also sheet 1
I13: JP3.28 U43.8(OUT) ; also sheet 1
I14: JP3.30 U58.8(OUT) ; also sheet 1
I15: JP3.32 U52.8(OUT) ; also sheet 1
M1I0: U48.2(IN) ; also sheet 1
M1I1: U45.2(IN) ; also sheet 1
M1I2: U53.2(IN) ; also sheet 1
M1I3: U44.2(IN) ; also sheet 1
M1I4: U46.2(IN) ; also sheet 1
M1I5: U12.2(IN) ; also sheet 1
M1I6: U4.2(IN) ; also sheet 1
M1I7: U3.2(IN) ; also sheet 1
M1I8: U22.2(IN) ; also sheet 1
M1I9: U18.2(IN) ; also sheet 1
M1I10: U57.2(IN) ; also sheet 1
M1I11: U50.2(IN) ; also sheet 1
M1I12: U51.2(IN) ; also sheet 1
M1I13: U43.2(IN) ; also sheet 1
M1I14: U58.2(IN) ; also sheet 1
M1I15: U52.2(IN) ; also sheet 1
M2I0: U11.2(IN) ; also sheet 1
M2I1: U15.2(IN) ; also sheet 1
M2I2: U14.2(IN) ; also sheet 1
M2I3: U13.2(IN) ; also sheet 1
M2I4: U54.2(IN) ; also sheet 1
M2I5: U40.2(IN) ; also sheet 1
M2I6: U47.2(IN) ; also sheet 1
M2I7: U55.2(IN) ; also sheet 1
M2I8: U19.2(IN) ; also sheet 1
M2I9: U16.2(IN) ; also sheet 1
M2I10: U17.2(IN) ; also sheet 1
M2I11: U20.2(IN) ; also sheet 1
M2I12: U56.2(IN) ; also sheet 1
M2I13: U49.2(IN) ; also sheet 1
M2I14: U42.2(IN) ; also sheet 1
M2I15: U41.2(IN) ; also sheet 1
N$14: IC2.1(A:I) JP2.1
N$15: U41.7(S/H*)
N$16: U52.1(VCC)
N$17: JP3.1 U11.8(OUT)
N$19: JP3.3 U15.8(OUT)
N$21: JP3.5 U14.8(OUT)
N$23: JP3.7 U13.8(OUT)
N$25: U40.7(S/H*)
N$26: JP3.17 U19.8(OUT)
N$27: JP3.19 U16.8(OUT)
N$30: U4.7(S/H*)
N$31: U49.5(VEE)
N$32: U4.1(VCC)
N$33: JP3.21 U17.8(OUT)
N$35: JP3.23 U20.8(OUT)
N$36: JP3.25 U56.8(OUT)
N$37: JP3.27 U49.8(OUT)
N$39: U4.5(VEE)
N$40: U3.1(VCC)
N$41: U3.7(S/H*)
N$43: U53.7(S/H*)
N$45: U44.7(S/H*)
N$47: U46.7(S/H*)
N$49: U12.1(VCC)
N$50: U12.7(S/H*)
N$51: U12.5(VEE)
N$54: U3.5(VEE)
N$55: U11.1(VCC)
N$56: U11.7(S/H*)
N$57: U42.7(S/H*)
N$58: U11.5(VEE)
N$59: U15.1(VCC)
N$60: U15.7(S/H*)
N$61: U52.7(S/H*)
N$62: U15.5(VEE)
N$63: U14.7(S/H*)
N$64: U52.5(VEE)
N$65: U49.7(S/H*)
N$66: U56.7(S/H*)
N$67: U54.7(S/H*)
N$68: U13.7(S/H*)
N$69: U58.1(VCC)
N$70: U55.7(S/H*)
N$71: U47.7(S/H*)
N$72: U20.7(S/H*)
N$73: JP3.9 U54.8(OUT)
N$74: JP3.11 U40.8(OUT)
N$75: JP3.13 U47.8(OUT)
N$76: JP3.15 U55.8(OUT)
N$77: U58.7(S/H*)
N$78: U17.7(S/H*)
N$80: U16.1(VCC)
N$81: U16.7(S/H*)
N$82: U58.5(VEE)
N$83: U16.5(VEE)
N$84: U19.1(VCC)
N$85: U19.7(S/H*)
N$86: U43.1(VCC)
N$87: U19.5(VEE)
N$88: JP3.29 U42.8(OUT)
N$89: JP3.31 U41.8(OUT)
N$90: U43.7(S/H*)
N$92: U43.5(VEE)
N$93: U51.1(VCC)
N$94: U51.7(S/H*)
N$96: U51.5(VEE)
N$97: U50.1(VCC)
N$98: U50.7(S/H*)
N$100: U50.5(VEE)
N$101: U57.1(VCC)
N$102: U57.7(S/H*)
N$104: U57.5(VEE)
N$105: U18.1(VCC)
N$106: U18.7(S/H*)
N$108: U18.5(VEE)
N$109: U22.1(VCC)
N$110: U22.7(S/H*)
N$112: U22.5(VEE)
STATUS: IC2.2(A:O) U45.7(S/H*) U48.7(S/H*)
Unconnected: IC2.3(B:I) IC2.4(B:O) IC2.5(C:I) IC2.6(C:O) IC2.8(D:O) IC2.9(D:I) IC2.10(E:O) IC2.11(E:I) IC2.12(F:O) IC2.13(F:I) U3.4(NC) U3.6(NC_2) U4.4(NC) U4.6(NC_2) U11.4(NC) U11.6(NC_2) U12.4(NC) U12.6(NC_2) U13.4(NC) U13.6(NC_2) U14.4(NC) U14.6(NC_2) U15.4(NC) U15.6(NC_2) U16.4(NC) U16.6(NC_2) U17.4(NC) U17.6(NC_2) U18.4(NC) U18.6(NC_2) U19.4(NC) U19.6(NC_2) U20.4(NC) U20.6(NC_2) U22.4(NC) U22.6(NC_2) U40.4(NC) U40.6(NC_2) U41.4(NC) U41.6(NC_2) U42.4(NC) U42.6(NC_2) U43.4(NC) U43.6(NC_2) U44.4(NC) U44.6(NC_2) U45.4(NC) U45.6(NC_2) U46.4(NC) U46.6(NC_2) U47.4(NC) U47.6(NC_2) U48.4(NC) U48.6(NC_2) U49.4(NC) U49.6(NC_2) U50.4(NC) U50.6(NC_2) U51.4(NC) U51.6(NC_2) U52.4(NC) U52.6(NC_2) U53.4(NC) U53.6(NC_2) U54.4(NC) U54.6(NC_2) U55.4(NC) U55.6(NC_2) U56.4(NC) U56.6(NC_2) U57.4(NC) U57.6(NC_2) U58.4(NC) U58.6(NC_2)

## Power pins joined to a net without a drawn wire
GND: IC2.7(P:GND)
VCC: IC2.14(P:VCC)

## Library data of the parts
ADC1-2 SUPPLY = pinhead:PINHD-1X2: PIN HEADER
C3 C4 = rcl:C-EU: CAPACITOR, European symbol; SPICEPREFIX: C
DEMUX3 DEMUX4 MUX1_2 = pinhead:PINHD-1X5: PIN HEADER
IC2 = 74xx-eu:74*04: Hex INVERTER
JP2 = pinhead:PINHD-1X1: PIN HEADER
JP3 = pinhead:PINHD-2X16: PIN HEADER
JP6 = pinhead:PINHD-2X8: PIN HEADER
R1-R122 R124 R125 = rcl:R-US_: RESISTOR, American symbol; SPICEPREFIX: R
U1 U2 U5-U8 U21 U23 U28-U39 U59-U88 = OPA657U:OPA657U; DESCRIPTION: 1.6GHz, Low Noise, FET-Input Operational Amplifier 8-SOIC -40 to 85; DIGI-KEY_PART_NUMBER: OPA657UB-ND; MF: Texas Instruments; MP: OPA657U; PACKAGE: SOIC-8 Texas Instruments; PURCHASE-URL: https://pricing.snapeda.com/search/part/OPA657U/?ref=eda
U3 U4 U11-U20 U22 U40-U58 = AD781JNZ:AD781JNZ: Sample and Hold Amplifier Check prices; AVAILABILITY: Good; DESCRIPTION: Sample and Hold Amplifier 1 Circuit 8-PDIP; MF: Analog Devices; MP: AD781JNZ; PACKAGE: PDIP-8 Analog Devices; PRICE: None; PURCHASE-URL: https://pricing.snapeda.com/search/part/AD781JNZ/?ref=eda
U9 U10 U26 U27 = CD74HCT4067M:CD74HCT4067M: Check prices; AVAILABILITY: Good; DESCRIPTION: 5-V, 16:1, 1-channel analog multiplexer with TTL inputs 24-SOIC -55 to 125; MF: Texas Instruments; MP: CD74HCT4067M; PACKAGE: SOIC-24 Texas Instruments; PRICE: None; PURCHASE-URL: https://pricing.snapeda.com/search/part/CD74HCT4067M/?ref=eda
U24 U25 = H11AA4SR2M:H11AA4SR2M: None Check prices; AVAILABILITY: Good; DESCRIPTION: Optoisolator Transistor with Base Output 4170Vrms 1 Channel 6-SMD; MF: ON Semiconductor; MP: H11AA4SR2M; PACKAGE: PDIP-6 ON Semiconductor; PRICE: None; PURCHASE-URL: https://pricing.snapeda.com/search/part/H11AA4SR2M/?ref=eda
